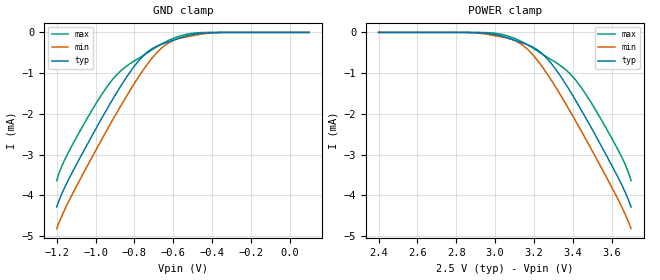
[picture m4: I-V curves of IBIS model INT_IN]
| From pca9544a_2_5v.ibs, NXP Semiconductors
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[Model]   INT_IN
Model_type Input
Vinh=2
Vinl=0.7
C_comp   0.5p   0.5p   0.5p
[Temperature Range] 27   85   -40
[Voltage Range]   2.5   2.25   2.75
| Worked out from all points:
|   GND clamp passes 1 mA (typ) near -0.83 V on its own axis
[GND Clamp]
-1.2V     -4.288mA   -4.821mA   -3.642mA
-1.17V    -3.927mA   -4.471mA   -3.246mA
-1.11V    -3.352mA   -3.889mA   -2.683mA
-1V       -2.383mA   -2.909mA   -1.767mA
-920mV    -1.713mA   -2.221mA   -1.203mA
-860mV    -1.243mA   -1.724mA   -901.9uA
-770mV    -654.5uA   -1.033mA   -614.4uA
-710mV    -405uA     -638uA     -431uA
-650mV    -271.1uA   -343.2uA   -260.8uA
-540mV    -96.45uA   -116.4uA   -55.76uA
-410mV    -6.277uA   -17.26uA   -938nA
100mV     774fA      7.819pA    302.5fA
[POWER Clamp]
2.4V      774fA      7.819pA    302.5fA
2.91V     -6.277uA   -17.26uA   -938nA
3.04V     -96.45uA   -116.4uA   -55.76uA
3.15V     -271.1uA   -343.2uA   -260.8uA
3.21V     -405uA     -638uA     -431uA
3.27V     -654.5uA   -1.033mA   -614.4uA
3.36V     -1.243mA   -1.724mA   -901.9uA
3.42V     -1.713mA   -2.221mA   -1.203mA
3.5V      -2.383mA   -2.909mA   -1.767mA
3.61V     -3.352mA   -3.889mA   -2.683mA
3.67V     -3.927mA   -4.471mA   -3.246mA
3.7V      -4.288mA   -4.821mA   -3.642mA
